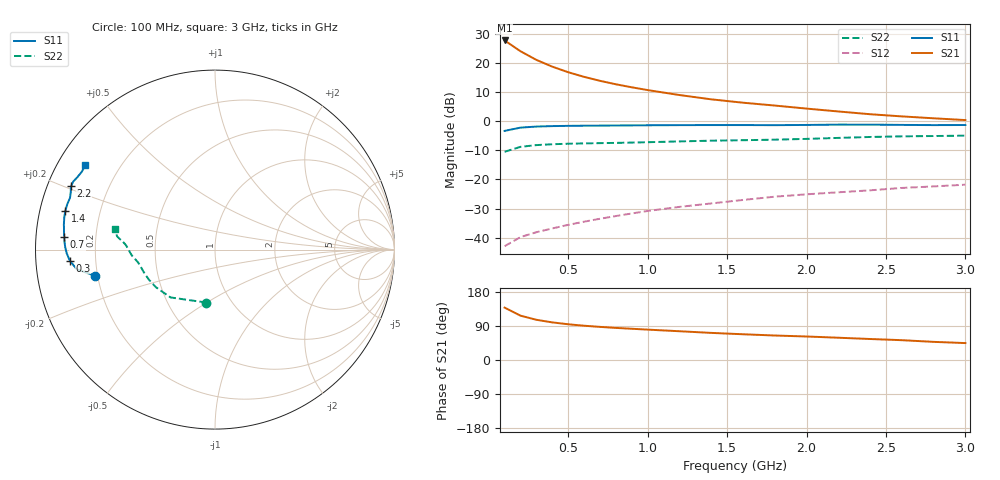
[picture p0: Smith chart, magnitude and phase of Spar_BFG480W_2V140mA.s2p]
! Filename: 2140BFG480.001
! Title: BFG480W
! Bias: Vce=2V; Ic=140mA
! Company: NXP Semiconductors NL
! User: Quality&Reliability T&D
! Measure time: 10 Nov 1999 / 11:55:48
#  MHz  S  MA  R 50
! Freq  S11  S21  S12  S22  :
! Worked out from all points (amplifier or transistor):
!   20 points, 100 MHz to 3 GHz, reference 50 ohm
!   highest |S21| = 27.8 dB at 100 MHz (marker M1)
!   |S21| within 3 dB of that: start of sweep to 180.9 MHz
!   unconditionally stable (mu >= 1): start of sweep to end of sweep
!   at 400 MHz: K = 1.34, MAG = 24.3 dB, |S12| = -36.8 dB
!   at 1.2 GHz: K = 1.49, MAG = 15.1 dB, |S12| = -29.4 dB
!   at 3 GHz: K = 1.51, MAG = 6.9 dB, |S12| = -21.8 dB
!   S11 on the Smith chart (normalised r, x): 100 MHz: 0.19, -0.10; 300 MHz: 0.10, -0.04; 700 MHz: 0.09, +0.04; 1.4 GHz: 0.08, +0.13; 2.2 GHz: 0.07, +0.21; 3 GHz: 0.08, +0.29
100  0.6838 -167.7  24.46 138.3  0.007155 58.1  0.2991 -99.2
200  0.778 -171.9  15.96 117.0  0.01026 53.4  0.3638 -132.9
300  0.8115 -175.7  11.34 106.1  0.01243 55.4  0.3898 -147.3
400  0.8263 -178.5  8.678 99.3  0.01443 58.7  0.4035 -155.0
500  0.8344 179.2  6.963 94.3  0.01662 61.8  0.4114 -159.7
600  0.8395 177.1  5.797 90.5  0.01885 64.1  0.417 -162.9
700  0.8427 175.3  4.957 87.4  0.02114 66.3  0.4212 -165.4
800  0.8465 173.6  4.323 84.7  0.02356 68.0  0.4255 -167.5
900  0.8497 172.0  3.836 82.4  0.02608 69.7  0.4308 -169.4
1000  0.8537 170.5  3.437 80.2  0.02876 70.7  0.437 -171.1
1200  0.859 167.8  2.825 75.9  0.03384 72.1  0.4512 -173.8
1400  0.8611 165.4  2.383 71.5  0.03878 72.7  0.464 -175.9
1600  0.8611 162.9  2.086 67.9  0.0445 73.1  0.4728 -177.9
1800  0.8578 160.3  1.863 64.6  0.05065 73.3  0.4834 179.6
2000  0.8648 158.3  1.652 62.0  0.05566 74.0  0.4983 176.9
2200  0.8766 156.3  1.475 58.8  0.06026 73.7  0.5181 174.8
2400  0.8762 154.4  1.322 55.4  0.06515 73.0  0.5375 173.4
2600  0.8667 152.3  1.213 52.3  0.0716 72.0  0.5511 172.3
2800  0.8595 149.7  1.126 47.9  0.07606 70.5  0.5581 170.6
3000  0.8629 147.1  1.049 44.7  0.08145 69.6  0.567 168.1
